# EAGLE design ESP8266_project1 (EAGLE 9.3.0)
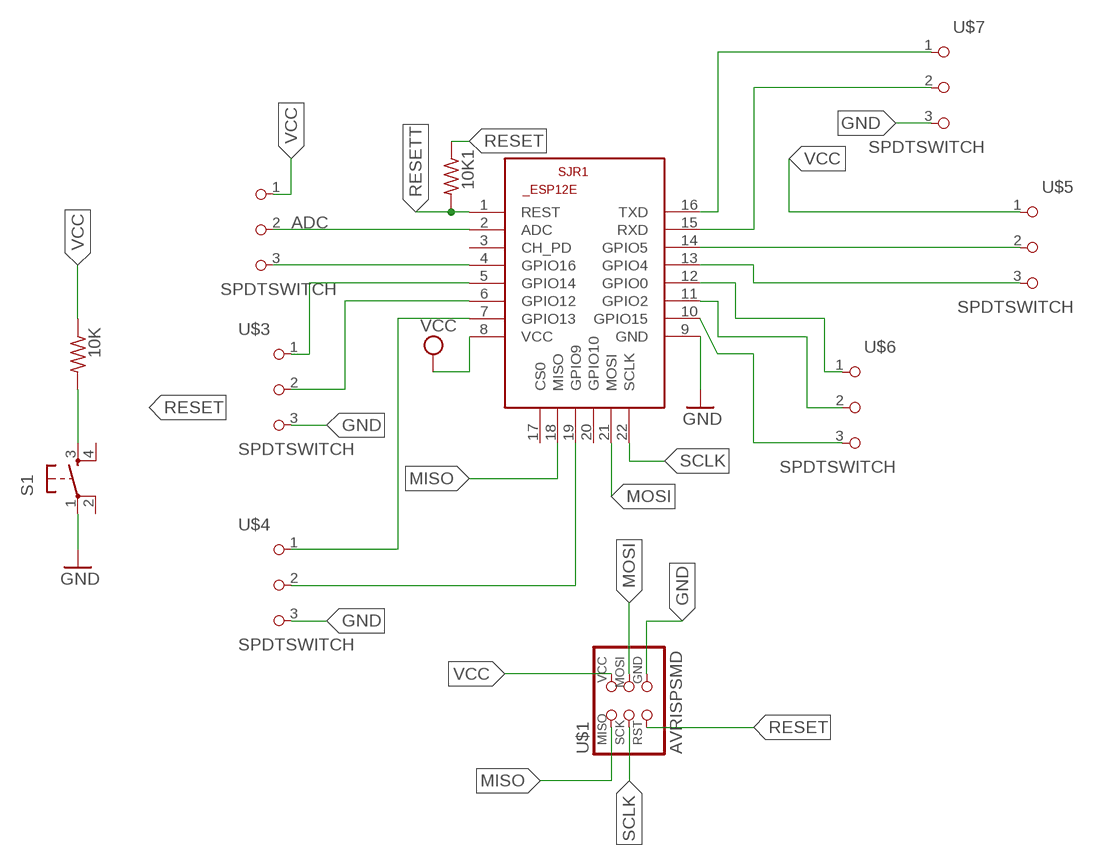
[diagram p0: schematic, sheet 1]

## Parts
10K  RES-US1206FAB  [R1206FAB]
10K1  RES-US1206FAB  [R1206FAB]
ADC  SPDTSWITCH  [SPDTSWITCH]
S1  6MM_SWITCH6MM_SWITCH  [6MM_SWITCH]
SJR1  ESP8266-12EESP12E  [ESP8266-ESP12E]
U$1  AVRISPSMD  [2X03SMD]
U$3  SPDTSWITCH  [SPDTSWITCH]
U$4  SPDTSWITCH  [SPDTSWITCH]
U$5  SPDTSWITCH  [SPDTSWITCH]
U$6  SPDTSWITCH  [SPDTSWITCH]
U$7  SPDTSWITCH  [SPDTSWITCH]

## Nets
4: SJR1.13(GPIO4) U$5.3
12: SJR1.6(GPIO12) U$3.2
14: SJR1.5(GPIO14) U$3.1
16: ADC.3 SJR1.4(GPIO16)
GND: S1.1(P) SJR1.9(GND) U$1.6(GND) U$3.3 U$4.3 U$7.3
MISO: SJR1.18(MISO) U$1.1(MISO)
MOSI: SJR1.21(MOSI) U$1.4(MOSI)
N$1: ADC.2 SJR1.2(ADC)
N$2: SJR1.19(GPIO9) U$4.2
N$3: SJR1.14(GPIO5) U$5.2
N$4: SJR1.7(GPIO13) U$4.1
N$5: SJR1.16(TXD) U$7.1
N$7: SJR1.12(GPIO0) U$6.1
N$9: SJR1.15(RXD) U$7.2
N$11: SJR1.11(GPIO2) U$6.2
N$12: SJR1.10(GPIO15) U$6.3
RESET: 10K1.1 10K.2 S1.3(S) U$1.5(RST)
RESETT: 10K1.2 SJR1.1(REST)
SCLK: SJR1.22(SCLK) U$1.3(SCK)
VCC: 10K.1 ADC.1 SJR1.8(VCC) U$1.2(VCC) U$5.1
Unconnected: S1.2(P1) S1.4(S1) SJR1.3(CH_PD) SJR1.17(CS0) SJR1.20(GPIO10)

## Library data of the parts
10K 10K1 = fab:RES-US: Resistor (US Symbol)
ADC U$3-U$7 = fab:SPDTSWITCH
S1 = fab:6MM_SWITCH: OMRON SWITCH
SJR1 = esp12e:ESP8266-12E: ESP8266-12E Library for Eagle CAD The author not responsible for any damages or errors!. Created by Suhail jr.lt;/author>
U$1 = fab:AVRISP

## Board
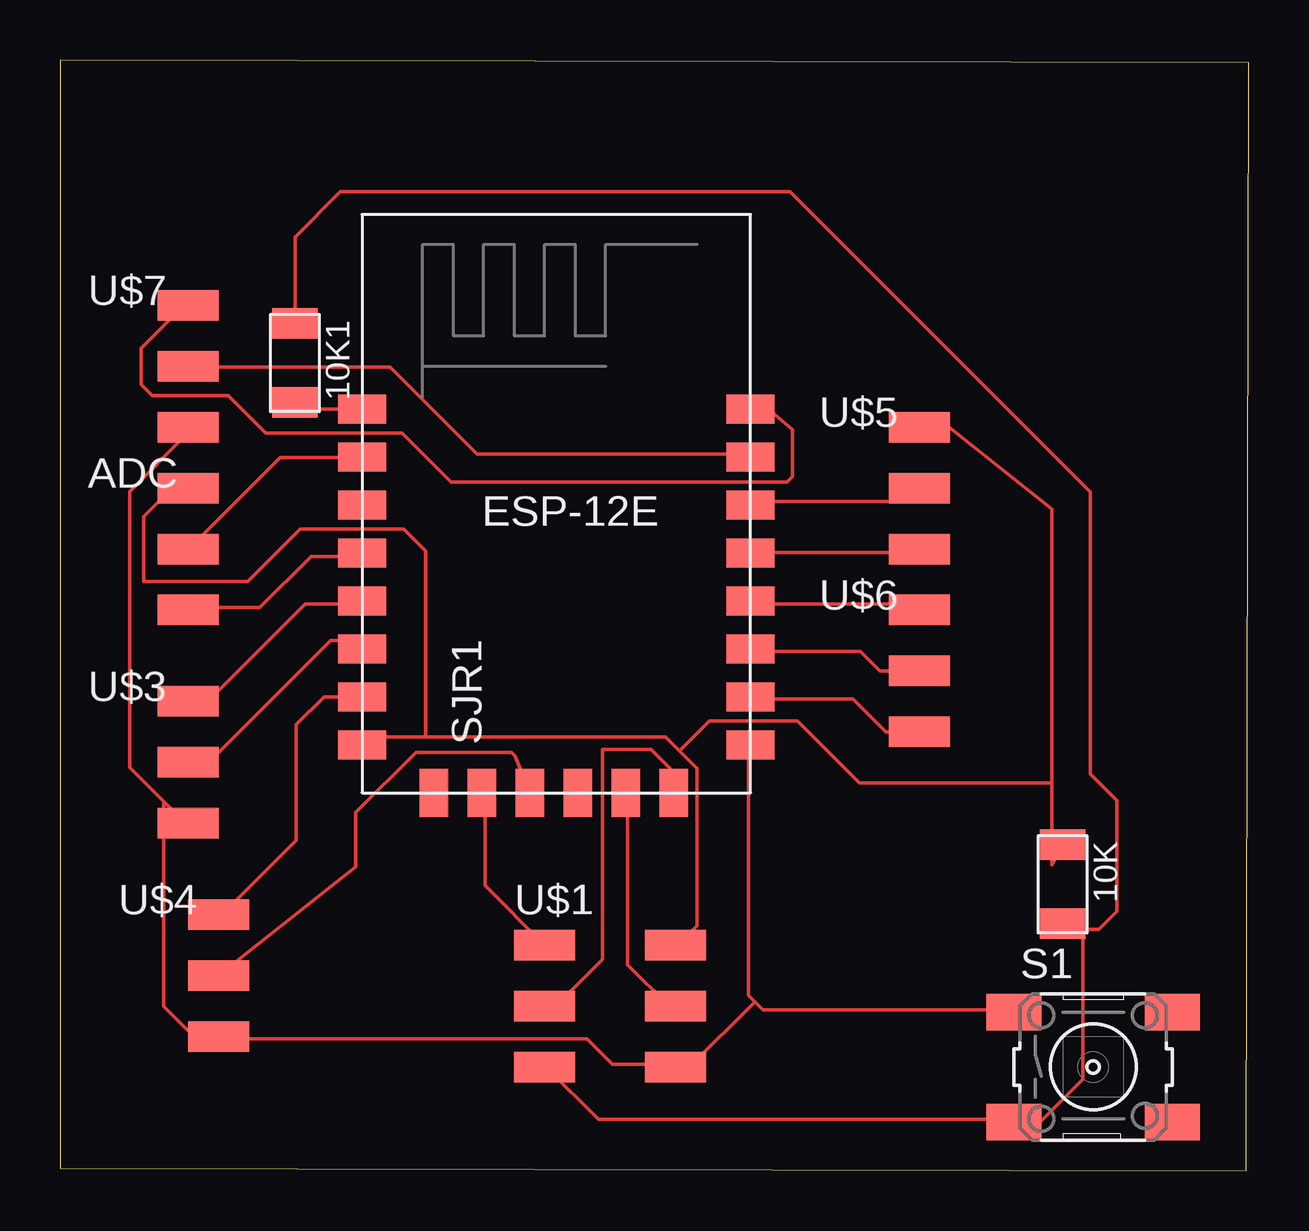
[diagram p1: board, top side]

Size 49.55 x 46.29 mm. Coordinates in mm from the lower left corner, seen from the top.
Outline: 0,0.1 49.44,0 49.55,46.19 0,46.29 0,0.1
Copper layers (1*16): Top 0.035mm / dielectric 1.5mm / Bottom 0.035mm
Design rules "default": minimum track width 6mil, minimum drill 0.35mm, track to track 6mil, track to pad 6mil, pad to pad 6mil, via to via 6mil, smd to smd 6mil, copper to edge 40mil, drill to drill 6mil, minimum pad ring 10mil, minimum via ring 8mil, stop-mask expansion 4mil, vias tented up to drill 0mil, thermal gap 10mil

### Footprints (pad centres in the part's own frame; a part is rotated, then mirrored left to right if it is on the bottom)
R1206FAB = smd 1.27 x 1.905: 1 -1.651,0; 2 1.651,0
SPDTSWITCH = smd 2.54 x 1.27: 1 0.38,2.54; 2 0.38,0; 3 0.38,-2.54
6MM_SWITCH = smd 2.286 x 1.524: 1 -3.302,2.286; 2 3.302,2.286; 3 -3.302,-2.286; 4 3.302,-2.286
ESP8266-ESP12E = smd 2 x 1.2: 1 -7.62,5.84; 2 -7.62,3.84; 3 -7.62,1.84; 4 -7.62,-0.16; 5 -7.62,-2.16; 6 -7.62,-4.16; 7 -7.62,-6.16; 8 -7.62,-8.16; 9 8.58,-8.16; 10 8.58,-6.16; 11 8.58,-4.16; 12 8.58,-2.16; 13 8.58,-0.16; 14 8.58,1.84; 15 8.58,3.84; 16 8.58,5.84 | smd 1.2 x 2: 17 -4.62,-10.16; 18 -2.62,-10.16; 19 -0.62,-10.16; 20 1.38,-10.16; 21 3.38,-10.16; 22 5.38,-10.16
2X03SMD = smd 2.54 x 1.27: 1 -2.54,2.54; 2 2.92,2.54; 3 -2.54,0; 4 2.92,0; 5 -2.54,-2.54; 6 2.92,-2.54

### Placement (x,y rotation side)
10K  41.79,11.94 270 top
10K1  9.79,33.66 270 top
ADC  4.96,25.91 0 top
S1  43.06,4.32 0 top
SJR1  20.2,25.91 0 top
U$1  22.74,6.86 0 top
U$3  4.96,17.02 0 top
U$4  6.23,8.13 0 top
U$5  35.44,28.45 0 top
U$6  35.44,20.83 0 top
U$7  4.96,33.53 0 top

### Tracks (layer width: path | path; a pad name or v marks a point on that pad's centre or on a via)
4
  Top 0.152: SJR1.13 28.84,25.75 35.7,25.75 35.8,25.86 U$5.3
12
  Top 0.152: U$3.2 6.2,17.02 11.28,22.1 12.08,22.1 SJR1.6
  Top 0.406: SJR1.6 12.23,22.1
14
  Top 0.152: U$3.1 6.15,19.56 10.21,23.62 12.53,23.62 SJR1.5
16
  Top 0.152: SJR1.4 12.53,25.6 10.46,25.6 8.32,23.47 5.37,23.47 ADC.3
GND
  Top 0.152: 28.69,17.37 28.69,17.68 SJR1.9 28.69,17.37 | 28.69,17.37 28.69,7.31 28.85,7.16 28.97,7.04 | 28.97,7.04 26.25,4.32 U$1.6 25.64,4.42 23.03,4.42 21.96,5.48 6.74,5.48 U$4.3 5.58,5.59 4.32,6.85 4.32,15.38 | 28.97,7.04 29.3,6.7 39.66,6.7 S1.1 | 4.32,15.38 5.22,14.48 U$3.3 | 4.32,15.38 2.9,16.8 2.9,28.31 5.22,30.63 5.22,30.94 U$7.3
MISO
  Top 0.152: U$1.1 17.71,11.89 17.71,15.7 SJR1.18
MOSI
  Top 0.152: SJR1.21 23.66,15.7 23.66,8.58 25.38,6.86 U$1.4
N$1
  Top 0.152: SJR1.2 12.53,29.72 9.18,29.72 5.37,25.91 ADC.2
N$2
  Top 0.152: SJR1.19 18.98,17.28 18.82,17.43 14.84,17.43 12.33,14.92 12.33,12.66 U$4.2
N$3
  Top 0.152: SJR1.14 28.84,27.89 35.24,27.89 35.8,28.45 U$5.2
N$4
  Top 0.152: SJR1.7 11.01,19.75 9.85,18.59 9.85,13.77 6.74,10.67 U$4.1
N$5
  Top 0.152: SJR1.16 29.54,31.75 30.52,30.89 30.52,28.93 30.3,28.71 16.3,28.71 14.26,30.75 8.58,30.75 7.02,32.31 3.85,32.31 3.39,32.76 3.39,34.29 5.22,36.12 U$7.1
N$7
  Top 0.152: SJR1.12 28.84,23.62 35.55,23.62 35.8,23.37 U$6.1
N$9
  Top 0.152: U$7.2 5.98,33.53 6.01,33.5 13.76,33.5 17.39,29.87 28.69,29.87 SJR1.15
N$11
  Top 0.152: U$6.2 34.17,20.83 33.36,21.64 28.84,21.64 SJR1.11
N$12
  Top 0.152: U$6.3 34.42,18.29 33.05,19.66 28.84,19.66 SJR1.10
RESET
  Top 0.152: 10K.2 41.99,10.06 42.44,10.06 | 39.81,2.13 S1.3 | 20.15,4.42 U$1.5 20.31,4.27 22.44,2.13 39.66,2.13 S1.3 | 10K1.1 9.79,38.91 11.68,40.8 30.44,40.8 42.95,28.29 42.95,16.53 44.05,15.42 44.05,10.81 43.3,10.06 42.44,10.06 | S1.3 40.87,2.03 42.64,3.81 42.64,9.86 42.44,10.06
RESETT
  Top 0.152: 12.53,31.85 SJR1.1 10.06,31.75 10K1.2
SCLK
  Top 0.152: SJR1.22 25.59,16.59 24.63,17.54 22.61,17.54 22.61,8.8 20.67,6.86 U$1.3
VCC
  Top 0.152: 41.34,16.15 41.34,27.58 37.04,30.99 U$5.1 | 41.34,16.15 41.34,12.73 10K.1 | 15.24,18.07 25.25,18.07 25.82,17.5 | 15.24,18.07 12.91,18.07 SJR1.8 | 25.82,17.5 26.1,17.22 26.55,16.76 26.55,10.21 25.79,9.45 U$1.2 | ADC.1 4.69,28.45 3.5,27.26 3.5,24.55 7.82,24.55 10.02,26.75 14.31,26.75 15.24,25.82 15.24,18.07 | 41.34,16.15 33.33,16.15 30.74,18.74 27.06,18.74 25.82,17.5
